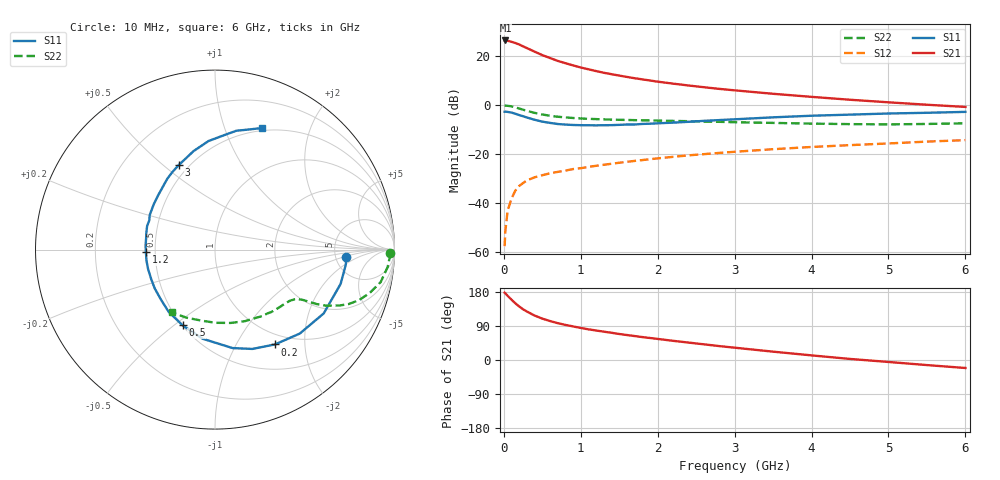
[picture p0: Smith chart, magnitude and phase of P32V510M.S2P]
! SIEMENS Small Signal Semiconductors
! BFP181
! Si NPN RF Bipolar Junction Transistor in SOT143
! VCE = 2.5 V  IC = 10 mA
! Common Emitter S-Parameters:  March  1996
# GHz  S  MA  R  50
!  f  S11  S21  S12  S22
! GHz  MAG  ANG  MAG  ANG  MAG  ANG  MAG  ANG
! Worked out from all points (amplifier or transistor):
!   36 points, 10 MHz to 6 GHz, reference 50 ohm
!   highest |S21| = 26.4 dB at 20 MHz (marker M1)
!   |S21| within 3 dB of that: start of sweep to 291.2 MHz
!   unconditionally stable (mu >= 1): 1.044 GHz to end of sweep
!   at 250 MHz: K = 0.36, MSG = 28.0 dB, |S12| = -31.9 dB
!   at 1.4 GHz: K = 1.12, MAG = 16.3 dB, |S12| = -24.0 dB
!   at 6 GHz: K = 1.01, MAG = 6.2 dB, |S12| = -14.3 dB
!   S11 on the Smith chart (normalised r, x): 10 MHz: 6.25, -1.13; 200 MHz: 0.84, -1.46; 500 MHz: 0.50, -0.54; 1.2 GHz: 0.44, -0.01; 3 GHz: 0.44, +0.56; 6 GHz: 0.47, +1.35
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0.01  0.7318 -3.3  20.9 177.6  0.0013 82.2  0.9766 -1.0
0.02  0.7336 -6.6  21 175.9  0.0027 82.0  0.9755 -2.2
0.05  0.7255 -15.3  20.67 169.2  0.007 87.8  0.9668 -5.8
0.1  0.7024 -30.4  19.72 159.1  0.0122 73.7  0.9406 -11.1
0.15  0.6649 -44.7  18.6 149.5  0.0179 68.4  0.8957 -15.6
0.2  0.6251 -57.7  17.36 141.2  0.0222 64.2  0.8509 -19.3
0.25  0.5913 -69.4  15.9 133.7  0.0254 60.2  0.8053 -22.1
0.3  0.5572 -79.9  14.66 127.9  0.0288 57.1  0.7622 -24.1
0.4  0.5013 -98.0  12.39 117.3  0.0333 52.9  0.6932 -26.8
0.5  0.4588 -113.2  10.53 109.2  0.0368 50.1  0.6421 -28.2
0.6  0.4322 -126.7  9.196 102.8  0.0403 49.0  0.6053 -28.9
0.7  0.41 -137.4  8.028 97.3  0.043 48.5  0.5781 -29.5
0.9  0.3918 -155.0  6.49 88.6  0.0491 48.2  0.5448 -30.6
1.1  0.3866 -171.0  5.402 80.9  0.0544 48.5  0.5232 -31.9
1.2  0.3852 -178.0  4.96 77.9  0.0573 48.4  0.5167 -32.8
1.7  0.4007 155.9  3.545 63.2  0.0721 48.4  0.4922 -38.0
2.2  0.4374 136.6  2.747 50.6  0.0873 46.7  0.4748 -44.7
3  0.5121 113.3  2.004 32.5  0.1108 42.0  0.4462 -57.8
3.5  0.5616 102.3  1.703 22.0  0.1252 38.7  0.432 -67.4
4.5  0.6382 85.7  1.286 2.8  0.1517 31.1  0.408 -89.4
5.5  0.6959 74.1  1.017 -13.4  0.1791 24.0  0.4113 -112.7
6  0.7262 68.9  0.917 -21.1  0.192 19.9  0.4242 -124.5
